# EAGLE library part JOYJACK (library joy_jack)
Joystick (Pin Header)
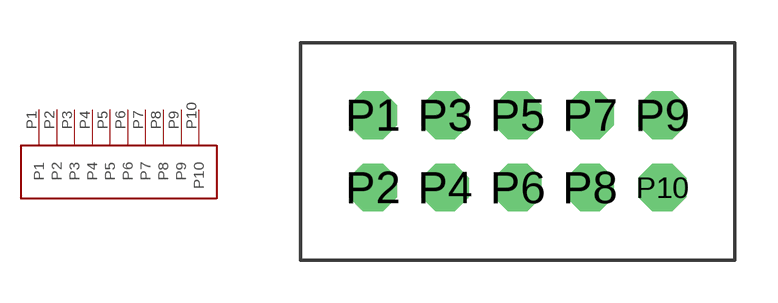
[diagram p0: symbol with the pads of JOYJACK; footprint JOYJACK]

Designator prefix -

## JOYJACK  [JOYJACK]
P1  P1
P2  P2
P3  P3
P4  P4
P5  P5
P6  P6
P7  P7
P8  P8
P9  P9
P10  P10

## Footprint JOYJACK (pad centres in mm)
Joystick (Pin Header)
drill 0.8 pad 1.676 octagon: P1 0,2.54; P2 0,0; P3 2.54,2.54; P4 2.54,0; P5 5.08,2.54; P6 5.08,0; P7 7.62,2.54; P8 7.62,0; P9 10.16,2.54; P10 10.16,0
